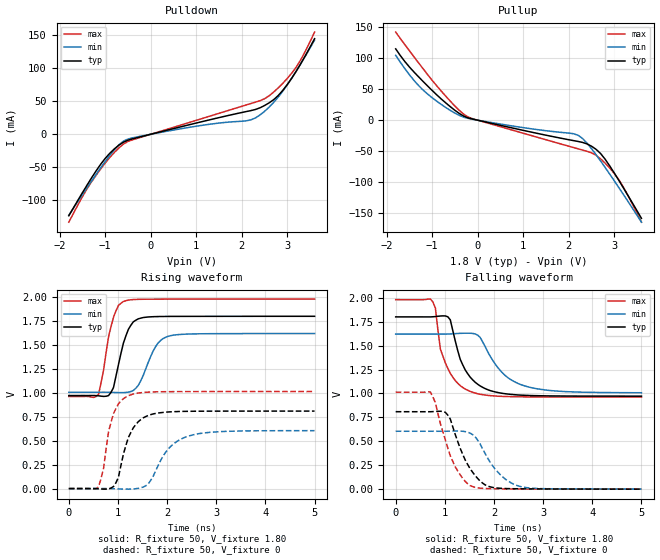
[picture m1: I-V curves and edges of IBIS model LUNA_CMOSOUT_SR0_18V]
[IBIS Ver]   3.2
[Comment Char]   |_char
[File name]   sg8201cga_18v_e.ibs
[File Rev]   1.1
[Date]   2021/10/19 9:35:58
[Source]
[Notes]
[Disclaimer]
This information is for modeling purposes only, and is not guaranteed.
Property of SEIKO EPSON Corp.,
unauthorized reproduction and/or distribution is strictly prohibited.
[Copyright]
Copyright 2021, SEIKO EPSON Corp.
[Component]   2G005_2016
Si_location Pin
Timing_location Pin
[Manufacturer]   SEIKO EPSON Corp.
| 2016 PKG
[Package]
R_pkg   42m   NA   NA
L_pkg   0.49n   NA   NA
C_pkg   0.178p   NA   NA
[Pin] signal_name   model_name
1   OE   NC
2   GND   GND
3   OUT   LUNA_CMOSOUT_SR0_18V
4   VCC   POWER
| Models and submodels in the file (1): LUNA_CMOSOUT_SR0_18V (Output)
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[Model]   LUNA_CMOSOUT_SR0_18V
Model_type Output
Polarity Non-Inverting
Vmeas=0.90
C_comp   2.5p   2.0p   3.0p
[Temperature Range] 25   140   -40
[Voltage Range]   1.80   1.62   1.98
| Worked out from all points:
|   slope of the pulldown table from 0 to 0.27 V, typ, clamps not added: 58.2 ohm
|   slope of the pullup table from 0 to 0.27 V, typ, clamps not added: 60.3 ohm
|   falling waveform, R_fixture 50, V_fixture 1.80: 20-80 % time 403ps typ, 579ps min, 334ps max; typ from 1.8 V to 0.972 V
|   falling waveform, R_fixture 50, V_fixture 0: 20-80 % time 424ps typ, 490ps min, 398ps max; typ from 0.81 V to 0.001 V
|   rising waveform, R_fixture 50, V_fixture 1.80: 20-80 % time 246ps typ, 319ps min, 223ps max; typ from 0.972 V to 1.8 V
|   rising waveform, R_fixture 50, V_fixture 0: 20-80 % time 304ps typ, 469ps min, 232ps max; typ from 0 V to 0.81 V
[Pullup]
-1.8V     114.9mA    104.4mA    141.9mA
-1.5V     85.82mA    73.36mA    112mA
-1.2V     62.58mA    48.66mA    83.04mA
-700mV    27.86mA    20.4mA     38.65mA
-300mV    6.361mA    4.687mA    9.35mA
-100mV    1.678mA    1.298mA    2.116mA
2.2V      -34.15mA   -23.98mA   -45.97mA
2.4V      -38.1mA    -36.68mA   -50.06mA
2.6V      -46.79mA   -55.35mA   -56.44mA
2.9V      -73.36mA   -86.58mA   -76.81mA
3.2V      -108.6mA   -119.3mA   -107.5mA
3.6V      -158.1mA   -164.2mA   -164.3mA
[Pulldown]
-1.8V     -123.7mA   -123mA     -133.5mA
-1.4V     -77.27mA   -81.17mA   -82.9mA
-1.1V     -45.54mA   -50.95mA   -52.73mA
-900mV    -28.87mA   -32.1mA    -35.22mA
-600mV    -12.08mA   -10.47mA   -14.92mA
800mV     13.67mA    9.961mA    16.89mA
2.1V      34.47mA    20.42mA    44.55mA
2.4V      40.15mA    29.22mA    50.94mA
2.8V      58.72mA    56.37mA    70.39mA
3.1V      85.32mA    85.42mA    92.99mA
3.3V      107.6mA    107.5mA    113.6mA
3.6V      145.2mA    143mA      155.1mA
[Falling Waveform]
R_fixture=50
V_fixture=1.80
V_fixture_min=1.62
V_fixture_max=1.98
0s        1.8V       1.62V      1.98V
757.6ps   1.801V     1.62V      1.954V
808.1ps   1.803V     1.62V      1.891V
909.1ps   1.809V     1.62V      1.465V
1.01ns    1.81V      1.62V      1.32V
1.111ns   1.769V     1.622V     1.21V
1.313ns   1.357V     1.628V     1.082V
1.515ns   1.171V     1.629V     1.022V
2.576ns   982mV      1.087V     964.8mV
5ns       972mV      1.008V     962.7mV
[Falling Waveform]
R_fixture=50
V_fixture=0
V_fixture_min=0
V_fixture_max=0
0s        809.6mV    605.4mV    1.014V
707.1ps   809.2mV    605.3mV    1.014V
808.1ps   812mV      605.2mV    902.4mV
1.061ns   773.7mV    606.1mV    429.4mV
1.212ns   570.6mV    608.4mV    233.8mV
1.515ns   213.5mV    585.7mV    37.36mV
1.869ns   34.19mV    327.1mV    6.503mV
2.172ns   8.522mV    130.9mV    3.358mV
2.475ns   4.534mV    37.55mV    2.228mV
5ns       763.6uV    1.441mV    443.9uV
[Rising Waveform]
R_fixture=50
V_fixture=1.80
V_fixture_min=1.62
V_fixture_max=1.98
0s        971.9mV    1.007V     962.7mV
606.1ps   969.1mV    1.007V     986mV
707.1ps   963mV      1.007V     1.237V
808.1ps   971.8mV    1.007V     1.586V
909.1ps   1.055V     1.005V     1.79V
1.111ns   1.521V     1.003V     1.955V
1.364ns   1.759V     1.048V     1.976V
1.768ns   1.797V     1.485V     1.979V
2.02ns    1.799V     1.591V     1.979V
5ns       1.8V       1.62V      1.98V
[Rising Waveform]
R_fixture=50
V_fixture=0
V_fixture_min=0
V_fixture_max=0
0s        18.6nV     512.3nV    17.1nV
606.1ps   -2.173mV   158.3uV    18.76mV
808.1ps   -3.873mV   -87.3uV    594.5mV
909.1ps   21.31mV    -1.67mV    783.3mV
1.01ns    119.3mV    -3.591mV   886.4mV
1.212ns   533.8mV    -6.063mV   970.5mV
1.616ns   764.3mV    50.02mV    1.008V
2.02ns    800.3mV    412mV      1.013V
2.424ns   807.2mV    547.3mV    1.013V
5ns       809.6mV    605.2mV    1.014V
[Ramp]
R_load=50
dV/dt_r   4.858E-1/3.039E-10   3.631E-1/4.664E-10   6.082E-1/2.298E-10
dV/dt_f   4.968E-1/4.028E-10   3.675E-1/5.774E-10   6.104E-1/3.335E-10
|[End   LUNA_CMOSOUT_SR0_18V
